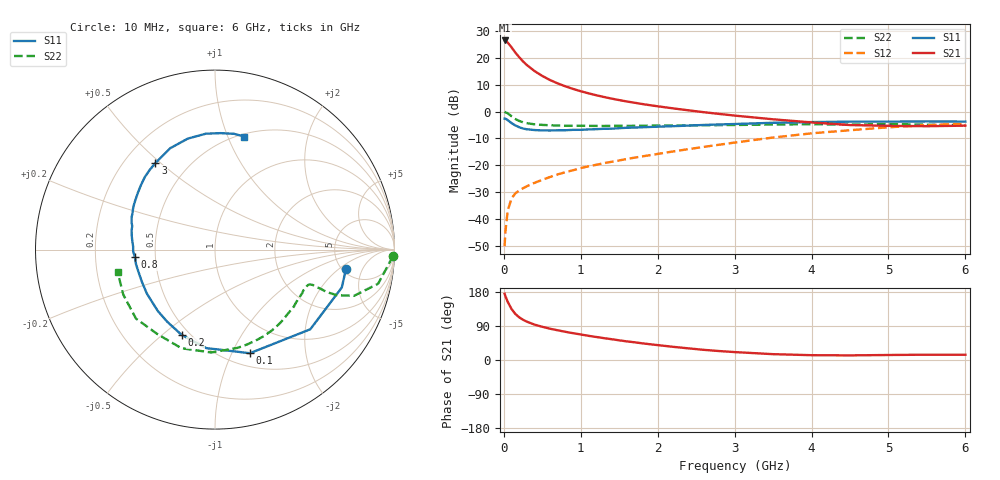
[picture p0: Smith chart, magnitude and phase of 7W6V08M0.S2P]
! Infineon Technologies  Discrete & RF Semiconductors
! BFS17W
! Si NPN RF Bipolar Junction Transistor in SOT323
! VCE = 6 V  IC = 8 mA
! Common Emitter S-Parameters:  August  1999
# GHz  S  MA  R  50
!  f  S11  S21  S12  S22
! GHz  MAG  ANG  MAG  ANG  MAG  ANG  MAG  ANG
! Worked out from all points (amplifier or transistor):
!   36 points, 10 MHz to 6 GHz, reference 50 ohm
!   highest |S21| = 26.5 dB at 10 MHz (marker M1)
!   |S21| within 3 dB of that: start of sweep to 111.1 MHz
!   unconditionally stable (mu >= 1): 466 MHz to 2.32 GHz; 5.213 GHz to end of sweep
!   at 250 MHz: K = 0.72, MSG = 23.6 dB, |S12| = -28.6 dB
!   at 1.4 GHz: K = 1.19, MAG = 9.1 dB, |S12| = -18.7 dB
!   at 6 GHz: K = 1.05, MAG = -1.7 dB, |S12| = -4.5 dB
!   S11 on the Smith chart (normalised r, x): 10 MHz: 5.42, -2.54; 100 MHz: 0.64, -1.18; 200 MHz: 0.45, -0.58; 800 MHz: 0.38, -0.04; 3 GHz: 0.33, +0.48; 6 GHz: 0.53, +1.15
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0.01  0.7381 -8.3  21.12 174.7  0.0031 82.7  0.9914 -2.1
0.02  0.7372 -16.7  20.85 168.9  0.0057 83.1  0.9689 -5.1
0.05  0.6921 -39.9  19.32 153.7  0.0142 71.4  0.9286 -11.8
0.1  0.6091 -71.4  15.71 134.6  0.0241 59.8  0.8162 -18.4
0.15  0.5508 -95.1  12.56 121.4  0.0299 55.1  0.7253 -20.5
0.2  0.5102 -111.4  10.28 112.6  0.0339 53.6  0.6685 -20.8
0.25  0.4819 -123.6  8.577 106.1  0.0372 52.5  0.6302 -20.4
0.3  0.4674 -133.0  7.338 101.1  0.0407 54.3  0.6069 -20.2
0.4  0.4519 -147.1  5.67 93.3  0.047 56.2  0.5775 -19.9
0.5  0.445 -156.5  4.605 87.6  0.0535 58.8  0.5638 -20.1
0.6  0.444 -163.6  3.866 82.6  0.0603 60.1  0.5549 -20.8
0.7  0.4475 -169.3  3.348 78.4  0.0674 62.2  0.5492 -22.0
0.8  0.4482 -174.6  2.952 74.4  0.0741 63.4  0.5451 -23.5
1.1  0.4639 173.7  2.186 63.8  0.0951 65.9  0.5406 -28.8
1.3  0.477 166.9  1.87 57.7  0.1093 67.0  0.5391 -33.1
1.6  0.4988 158.5  1.538 49.1  0.1307 68.6  0.5405 -39.8
2.2  0.5338 143.6  1.146 34.8  0.1804 70.6  0.5508 -55.1
3  0.5855 124.5  0.841 20.9  0.2642 69.0  0.5617 -77.1
3.5  0.6175 113.8  0.717 15.4  0.328 65.5  0.5736 -92.1
4.5  0.6478 94.5  0.56 12.2  0.4484 53.5  0.5697 -124.3
5.5  0.6538 80.6  0.533 14.0  0.5552 40.4  0.5693 -153.9
6  0.6503 75.4  0.546 13.9  0.5974 33.9  0.5567 -167.2
